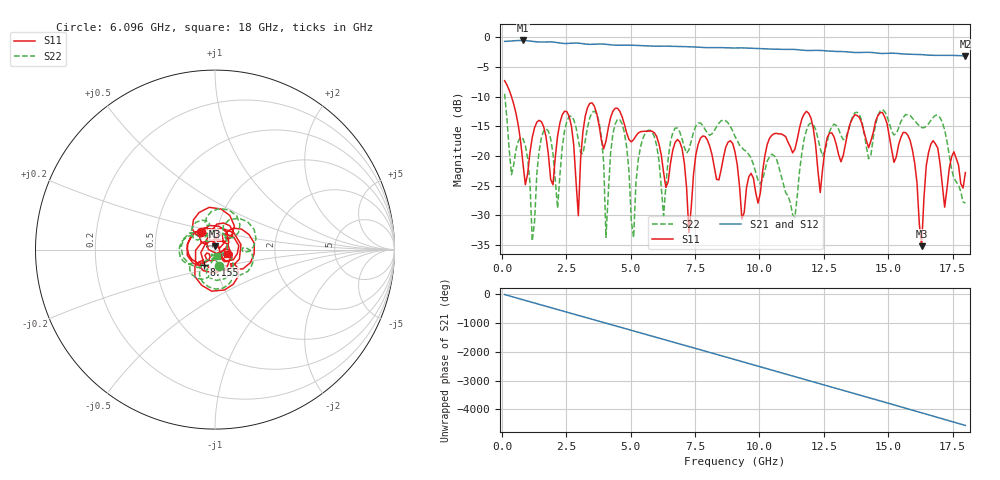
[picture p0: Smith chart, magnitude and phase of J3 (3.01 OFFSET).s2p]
!Agilent Technologies,E8364B,MY43040528,A.07.50.67
!Agilent E8364B: A.07.50.67
!Date: Wednesday, May 04, 2022 12:41:52
!Correction: S11(Full 2 Port(1,2))
!S21(Full 2 Port(1,2))
!S12(Full 2 Port(1,2))
!S22(Full 2 Port(1,2))
!S2P File: Measurements: S11, S21, S12, S22:
# Hz S  dB  R 50
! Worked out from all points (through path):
!   201 points, 100 MHz to 18 GHz, reference 50 ohm
!   highest |S21| = -0.56 dB at 816 MHz (marker M1); lowest = -3.2 dB at 18 GHz (marker M2)
!   group delay of S21, straight-line fit = 702 ps
!   lowest |S11| = -35.2 dB at 16.3 GHz (marker M3), VSWR 1.04, Z = 50.1 + j1.74 ohm
!   |S11| at or under -10 dB: 366.8 MHz to end of sweep
!   |S22| runs from -34.3 to -9.5 dB; largest |S21 - S12| = 0.013
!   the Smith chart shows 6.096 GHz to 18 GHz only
!   S11 on the Smith chart (normalised r, x): 6.096 GHz: 0.84, +0.17; 8.155 GHz: 0.88, -0.15; 18 GHz: 1.15, -0.05
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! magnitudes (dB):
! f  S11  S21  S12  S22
! 100 MHz  -7.3  -0.7  -0.6  -9.5
! 816 MHz  -21.4  -0.6  -0.5  -17.1
! 1.174 GHz  -16.9  -0.7  -0.6  -34.3
! 1.621 GHz  -15.1  -0.8  -0.8  -15.7
! 2.159 GHz  -16.6  -0.9  -0.9  -28.8
! 2.606 GHz  -13.3  -1.0  -1.0  -13.4
! 2.964 GHz  -30.1  -1.0  -1.0  -17.3
! 3.143 GHz  -15.9  -1.1  -1.0  -19.6
! 3.769 GHz  -14.8  -1.2  -1.1  -14.3
! 4.038 GHz  -17.5  -1.2  -1.1  -33.7
! 4.486 GHz  -12.0  -1.4  -1.3  -13.8
! 5.112 GHz  -17.2  -1.4  -1.3  -33.7
! 6.096 GHz  -18.0  -1.5  -1.5  -20.8
! 7.26 GHz  -32.9  -1.6  -1.5  -19.0
! 8.155 GHz  -19.8  -1.8  -1.7  -16.3
! 9.05 GHz  -19.3  -1.8  -1.8  -16.7
! 11.38 GHz  -18.9  -2.1  -2.0  -30.3
! 12.09 GHz  -15.4  -2.2  -2.2  -14.7
! 15.05 GHz  -16.8  -2.7  -2.7  -14.5
! 16.3 GHz  -35.2  -2.9  -2.9  -15.2
! 16.66 GHz  -18.0  -3.1  -3.0  -14.0
! 18 GHz  -22.8  -3.2  -3.1  -27.9
